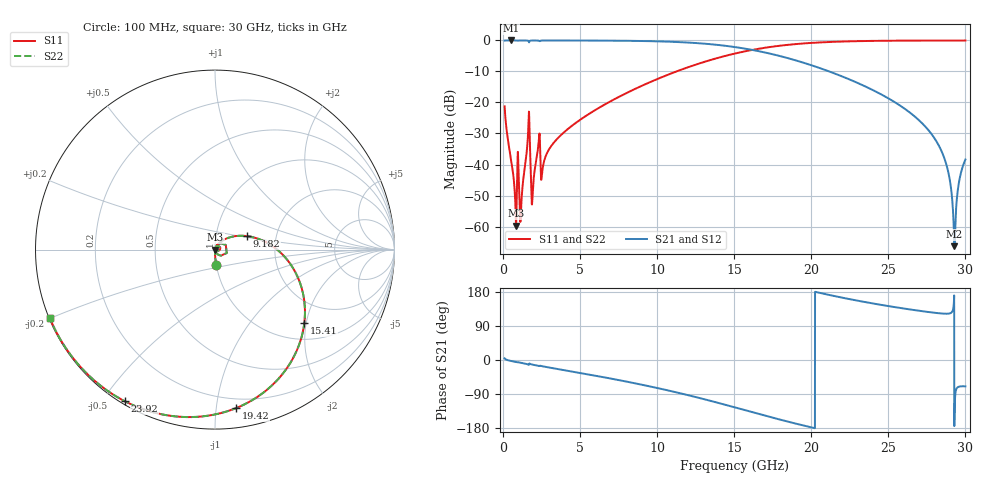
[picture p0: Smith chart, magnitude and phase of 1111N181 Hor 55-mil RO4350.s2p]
# GHz S MA R 50
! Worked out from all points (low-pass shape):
!   3201 points, 100 MHz to 30 GHz, reference 50 ohm
!   highest |S21| = -0.01 dB at 520.5 MHz (marker M1); lowest = -66.3 dB at 29.29 GHz (marker M2)
!   |S21| within 3 dB of the highest: start of sweep to 16.12 GHz
!   lowest |S11| = -59.7 dB at 847.5 MHz (marker M3), VSWR 1.00, Z = 50.1 - j0.0153 ohm
!   |S11| at or under -10 dB: start of sweep to 11.25 GHz
!   |S22| runs from -59.7 to 0.0 dB; largest |S21 - S12| = 0
!   S11 on the Smith chart (normalised r, x): 100 MHz: 1.00, -0.17; 9.182 GHz: 1.42, +0.22; 15.41 GHz: 1.39, -1.95; 19.42 GHz: 0.13, -1.13; 23.92 GHz: 0.01, -0.57; 30 GHz: 0.00, -0.20
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0.1  0.08666 -85.5  0.996 4.3  0.996 4.3  0.08666 -85.5
0.5204688  0.01206 -90.5  0.9994 -2.6  0.9994 -2.6  0.01206 -90.5
0.8475  0.001036 -8.5  0.9989 -5.4  0.9989 -5.4  0.001036 -8.5
1.202562  0.002791 61.6  0.9989 -7.8  0.9989 -7.8  0.002791 61.6
1.613687  0.02908 63.0  0.9918 -11.8  0.9918 -11.8  0.02908 63.0
1.940719  0.004242 53.8  0.9981 -12.5  0.9981 -12.5  0.004242 53.8
2.26775  0.01837 62.3  0.9956 -15.3  0.9956 -15.3  0.01837 62.3
2.576094  0.008833 59.4  0.9976 -16.7  0.9976 -16.7  0.008833 59.4
5.089563  0.05446 53.9  0.9967 -34.8  0.9967 -34.8  0.05446 53.9
9.182125  0.1945 22.7  0.9778 -66.7  0.9778 -66.7  0.1945 22.7
10.06978  0.2422 15.0  0.9668 -74.5  0.9668 -74.5  0.2422 15.0
15.05  0.6154 -35.5  0.7821 -125.1  0.7821 -125.1  0.6154 -35.5
15.40506  0.6442 -39.4  0.7585 -129.1  0.7585 -129.1  0.6442 -39.4
19.42288  0.8913 -82.5  0.4431 -172.2  0.4431 -172.2  0.8913 -82.5
20.03956  0.9134 -88.5  0.3959 -178.1  0.3959 -178.1  0.9134 -88.5
23.91722  0.9829 -120.7  0.162 149.8  0.162 149.8  0.9829 -120.7
25.01978  0.9895 -128.4  0.1158 142.2  0.1158 142.2  0.9895 -128.4
28.23403  0.9962 -148.1  0.02111 123.6  0.02111 123.6  0.9962 -148.1
28.87875  0.9964 -151.6  0.00776 122.3  0.00776 122.3  0.9964 -151.6
29.28987  0.9964 -153.8  0.0004826 -155.3  0.0004826 -155.3  0.9964 -153.8
29.63559  0.9964 -155.7  0.006063 -69.9  0.006063 -69.9  0.9964 -155.7
30  0.9963 -157.5  0.01203 -69.5  0.01203 -69.5  0.9963 -157.5
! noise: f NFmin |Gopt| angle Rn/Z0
0.1  0.0006799  0.7393  0.8642  0.0005221
3.417  0.008827  0.4381  20.95  0.002528
6.743  0.01481  0.3803  38.63  0.003465
10.06  0.02216  0.3964  53.7  0.004922
13.39  0.03254  0.4594  67.83  0.007398
16.7  0.0497  0.5661  83.25  0.01224
20.03  0.08369  0.7025  101.2  0.02323
23.35  0.1677  0.8366  120.6  0.05464
26.67  0.5083  0.9423  139.7  0.2353
30  2.532  0.9876  157.5  1.884
